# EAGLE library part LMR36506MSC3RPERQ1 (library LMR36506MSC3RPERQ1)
Buck Switching Regulator IC Positive Fixed 3.3V 1 Output 600mA 9-VFQFN Source: Datasheet
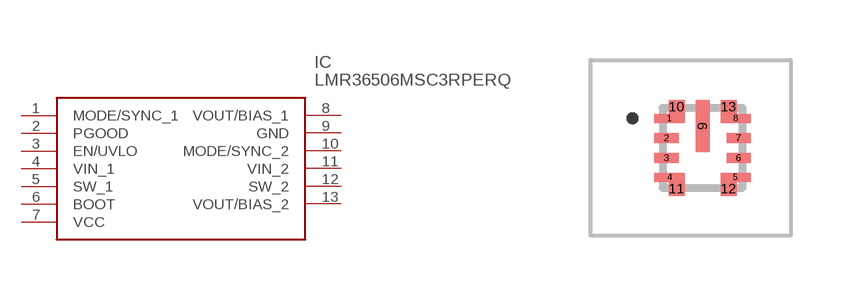
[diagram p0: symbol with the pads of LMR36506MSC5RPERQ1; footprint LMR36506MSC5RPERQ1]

Designator prefix IC

## LMR36506MSC3RPERQ1 (Description: Buck Switching Regulator IC Positive Fixed 3.3V 1 Output 600mA 9-VFQFN; Height: 1mm; Manufacturer_Name: Texas Instruments; Manufacturer_Part_Number: LMR36506MSC3RPERQ1; Mouser_Part_Number: 595-R36506MSC3RPERQ1; Mouser_Price-Stock: https://www.mouser.co.uk/ProductDetail/Texas-Instruments/LMR36506MSC3RPERQ1?qs=sPbYRqrBIVmjGKIOaXZOhA%3D%3D)  [LMR36506MSC5RPERQ1]
1  MODE/SYNC_1
2  PGOOD
3  EN/UVLO
4  VIN_1
5  SW_1
6  BOOT
7  VCC
8  VOUT/BIAS_1
9  GND
10  MODE/SYNC_2
11  VIN_2
12  SW_2
13  VOUT/BIAS_2

## Footprint LMR36506MSC5RPERQ1 (pad centres in mm)
RPE0009A
smd 0.75 x 0.225: 1 -0.825,0.738; 4 -0.825,-0.738; 5 0.825,-0.738; 8 0.825,0.738
smd 0.6 x 0.25: 2 -0.9,0.25; 3 -0.9,-0.25; 6 0.9,-0.25; 7 0.9,0.25
smd 0.35 x 1.3: 9 0,0.55
smd 0.4 x 0.35: 10 -0.65,1.026; 11 -0.65,-1.026; 12 0.65,-1.026; 13 0.65,1.026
